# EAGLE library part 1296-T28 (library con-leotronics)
1.27mm SINGLE ROW FEMALE SOCKET Source: http://www.leotronics.co.uk/Conexcon/Data%20Sheets/sec.%20A/1296ing.pdf
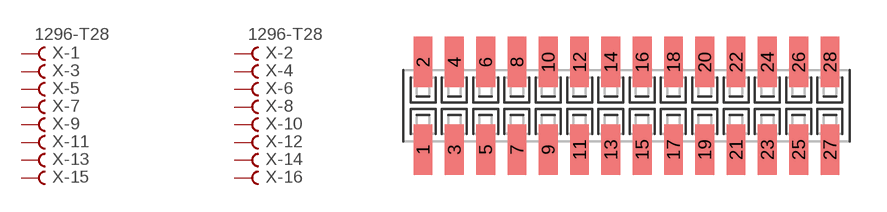
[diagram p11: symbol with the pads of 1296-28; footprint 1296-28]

Designator prefix X; gates -1=FVAL -2=FVAL -3=F -4=F -5=F -6=F -7=F -8=F -9=F -10=F -11=F -12=F -13=F -14=F -15=F -16=F -17=F -18=F -19=F -20=F -21=F -22=F -23=F -24=F -25=F -26=F -27=F -28=F

## 1296-T28 (OC_FARNELL: unknown; OC_NEWARK: unknown)  [1296-28]
1  -1:B  pas
2  -2:B  pas
3  -3:B  pas
4  -4:B  pas
5  -5:B  pas
6  -6:B  pas
7  -7:B  pas
8  -8:B  pas
9  -9:B  pas
10  -10:B  pas
11  -11:B  pas
12  -12:B  pas
13  -13:B  pas
14  -14:B  pas
15  -15:B  pas
16  -16:B  pas
17  -17:B  pas
18  -18:B  pas
19  -19:B  pas
20  -20:B  pas
21  -21:B  pas
22  -22:B  pas
23  -23:B  pas
24  -24:B  pas
25  -25:B  pas
26  -26:B  pas
27  -27:B  pas
28  -28:B  pas

## Footprint 1296-28 (pad centres in mm)
1.27mm SINGLE ROW FEMALE SOCKET Source: http://www.leotronics.co.uk/Conexcon/Data%20Sheets/sec.%20A/1296ing.pdf
smd 0.76 x 2.05: 1 -8.255,-1.78; 2 -8.255,1.78; 3 -6.985,-1.78; 4 -6.985,1.78; 5 -5.715,-1.78; 6 -5.715,1.78; 7 -4.445,-1.78; 8 -4.445,1.78; 9 -3.175,-1.78; 10 -3.175,1.78; 11 -1.905,-1.78; 12 -1.905,1.78; 13 -0.635,-1.78; 14 -0.635,1.78; 15 0.635,-1.78; 16 0.635,1.78; 17 1.905,-1.78; 18 1.905,1.78; 19 3.175,-1.78; 20 3.175,1.78; 21 4.445,-1.78; 22 4.445,1.78; 23 5.715,-1.78; 24 5.715,1.78; 25 6.985,-1.78; 26 6.985,1.78; 27 8.255,-1.78; 28 8.255,1.78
